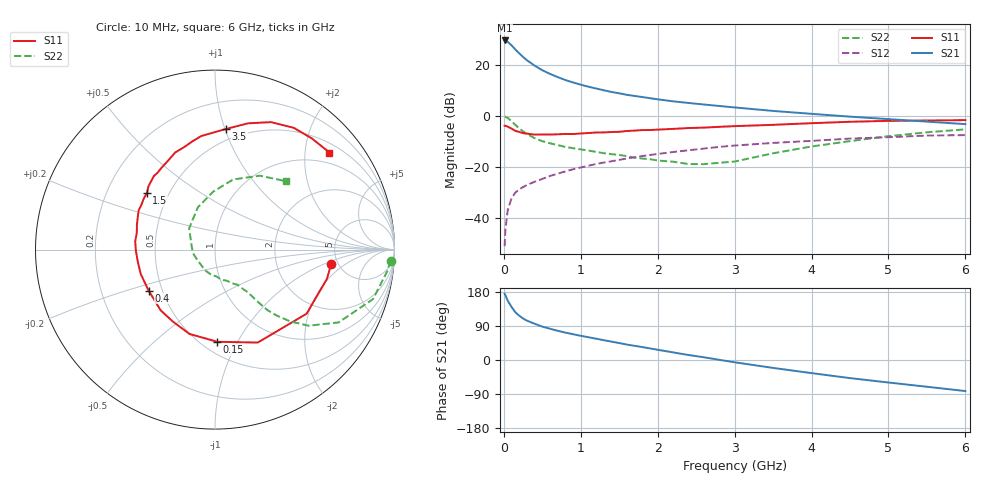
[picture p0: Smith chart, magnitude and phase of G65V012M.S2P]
! SIEMENS Small Signal Semiconductors
! BFG193
! Si NPN RF Bipolar Junction Transistor in SOT223
! VCE = 5 V  IC = 12 mA
! Common Emitter S-Parameters:  August  1996
# GHz  S  MA  R  50
!  f  S11  S21  S12  S22
! GHz  MAG  ANG  MAG  ANG  MAG  ANG  MAG  ANG
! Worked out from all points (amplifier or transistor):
!   36 points, 10 MHz to 6 GHz, reference 50 ohm
!   highest |S21| = 29.7 dB at 10 MHz (marker M1)
!   |S21| within 3 dB of that: start of sweep to 132.9 MHz
!   unconditionally stable (mu >= 1): 837.3 MHz to 2.468 GHz
!   at 250 MHz: K = 0.59, MSG = 25.5 dB, |S12| = -27.9 dB
!   at 1.4 GHz: K = 1.06, MAG = 12.1 dB, |S12| = -17.7 dB
!   at 6 GHz: K = 0.87, MSG = 2.2 dB, |S12| = -7.5 dB
!   S11 on the Smith chart (normalised r, x): 10 MHz: 4.37, -1.24; 150 MHz: 0.59, -0.83; 400 MHz: 0.42, -0.24; 1.5 GHz: 0.38, +0.31; 3.5 GHz: 0.41, +1.01; 6 GHz: 0.71, +2.55
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0.01  0.6519 -7.2  30.65 174.9  0.0028 95.6  0.9805 -3.6
0.02  0.6446 -14.7  30.33 171.0  0.0058 83.9  0.967 -7.2
0.05  0.6229 -35.0  28.76 156.8  0.0141 73.4  0.9225 -17.4
0.1  0.5701 -65.3  24.62 140.1  0.0244 64.9  0.7994 -30.5
0.15  0.5136 -88.6  20.32 125.9  0.0316 57.3  0.6723 -39.1
0.2  0.4909 -106.9  17.13 116.9  0.0365 55.1  0.579 -43.7
0.25  0.4645 -120.5  14.5 109.5  0.0405 53.2  0.5004 -47.0
0.3  0.4539 -131.9  12.54 103.9  0.0444 53.4  0.4485 -49.0
0.4  0.4346 -148.3  9.821 95.6  0.0515 53.0  0.3703 -50.8
0.5  0.4356 -161.7  7.977 88.1  0.0586 53.3  0.3225 -51.8
0.6  0.4354 -171.0  6.761 82.5  0.0668 53.7  0.2935 -52.8
0.7  0.4405 -178.9  5.847 77.1  0.0743 54.0  0.27 -54.6
0.9  0.4454 168.1  4.584 68.0  0.0907 53.0  0.2342 -57.1
1.1  0.4663 157.4  3.783 60.0  0.1064 51.9  0.2107 -63.2
1.5  0.4928 140.4  2.809 44.7  0.1386 46.6  0.1728 -77.5
1.7  0.5202 133.4  2.492 37.4  0.1562 43.7  0.1529 -84.7
2.2  0.5622 117.3  1.955 20.1  0.1977 34.4  0.1277 -116.5
2.8  0.6172 101.5  1.585 0.5  0.2491 22.2  0.1214 -167.4
3.5  0.6753 84.7  1.267 -20.9  0.2981 6.1  0.1866 140.6
4.5  0.7756 66.3  0.978 -47.8  0.3627 -13.7  0.3233 91.7
5.5  0.8215 48.9  0.781 -70.6  0.416 -37.7  0.4814 58.8
6  0.8361 40.3  0.698 -82.0  0.424 -51.6  0.5508 43.7
